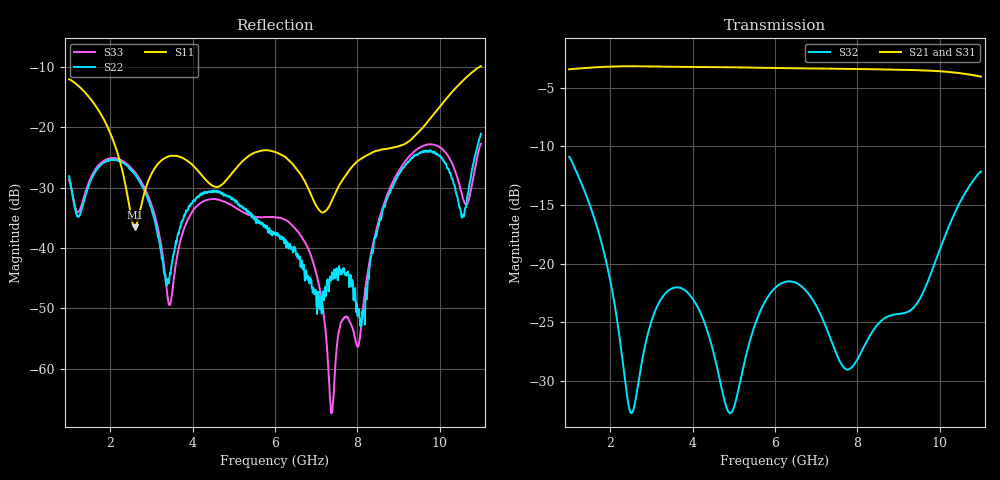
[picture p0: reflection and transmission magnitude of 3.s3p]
!The following data was pulled from an Agilent PNA
!This sNp file was generated from the data in the RF Test software
!NOTE:  Smoothing/Math/Corrections applied on any given trace ARE included in the data saved here
# MHz S dB R 50
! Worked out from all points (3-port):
!   1601 points, 1 GHz to 11 GHz, reference 50 ohm
!   strongest paths, dB at 1 GHz, 3.5 GHz, 6 GHz, 8.5 GHz, 11 GHz:
!     S21: -3.4, -3.2, -3.3, -3.4, -4.0
!     S31: -3.4, -3.2, -3.3, -3.5, -4.1
!     S32: -10.9, -22.1, -22.1, -25.2, -12.1
!   lowest |S11| = -36.6 dB at 2.594 GHz (marker M1), VSWR 1.03, Z = 48.9 + j0.964 ohm
!   |S11| at or under -10 dB: start of sweep to 10.96 GHz
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1000  -12.03 131.1  -3.41 -64.6  -3.43 -63.9
      -3.42 -63.7  -28.10 20.9  -10.89 -85.8
      -3.44 -63.9  -10.88 -85.8  -28.68 15.8
2593.75  -36.57 138.4  -3.16 -169.6  -3.18 -170.0
         -3.16 -169.6  -27.74 116.1  -32.02 -72.9
         -3.17 -170.0  -32.01 -72.8  -27.41 117.9
3437.5  -24.76 179.1  -3.20 133.8  -3.22 133.3
        -3.20 133.8  -44.90 -58.5  -22.24 -74.1
        -3.22 133.3  -22.24 -74.0  -49.45 -30.3
4168.75  -27.52 168.8  -3.22 84.6  -3.24 84.0
         -3.23 84.5  -31.27 -168.4  -24.04 -110.3
         -3.25 84.0  -24.04 -110.3  -32.66 -173.2
6000  -24.09 -163.4  -3.31 -40.8  -3.33 -41.6
      -3.31 -40.8  -37.56 -19.7  -22.09 -81.1
      -3.33 -41.7  -22.08 -81.1  -34.90 -34.6
6931.25  -32.02 -166.0  -3.35 -105.7  -3.38 -106.7
         -3.35 -105.8  -46.59 -167.6  -23.18 -126.3
         -3.37 -106.7  -23.17 -126.3  -42.48 -122.8
7375  -32.23 -106.3  -3.37 -137.1  -3.39 -138.1
      -3.38 -137.1  -45.30 77.9  -26.68 -134.1
      -3.39 -138.1  -26.66 -134.1  -67.38 -69.4
8137.5  -25.00 -95.4  -3.40 168.4  -3.43 167.2
        -3.40 168.3  -51.09 101.3  -27.25 -99.9
        -3.43 167.2  -27.25 -99.9  -49.85 178.6
9200  -22.55 -86.2  -3.47 90.8  -3.52 89.5
      -3.47 90.8  -25.97 70.6  -24.17 -104.9
      -3.52 89.5  -24.16 -105.0  -25.31 70.9
11000  -9.86 -110.9  -4.03 -44.6  -4.10 -47.3
       -4.04 -45.6  -21.06 142.0  -12.15 -141.2
       -4.10 -47.3  -12.15 -141.2  -22.73 146.2
